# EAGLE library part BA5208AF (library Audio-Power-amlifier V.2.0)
3V-400mW BTL Power Audio Amplifier
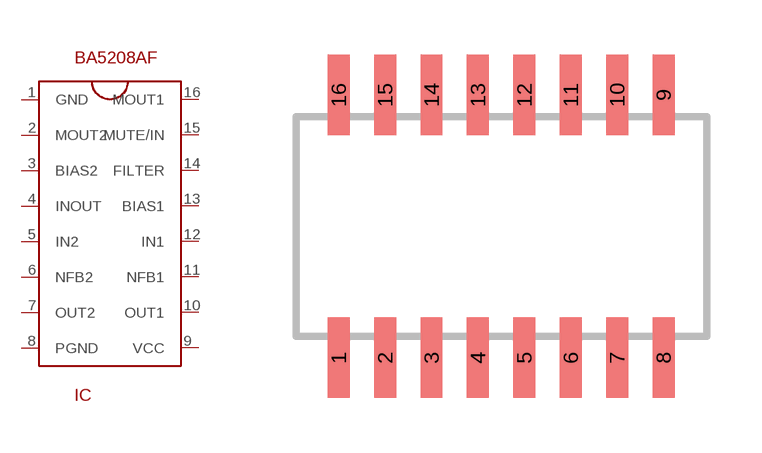
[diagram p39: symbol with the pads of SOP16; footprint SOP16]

Designator prefix IC

## BA5208AF  [SOP16]
1  GND  pwr
2  MOUT2  out
3  BIAS2
4  INOUT  out
5  IN2  in
6  NFB2
7  OUT2  out
8  PGND  pwr
9  VCC  pwr
10  OUT1  out
11  NFB1
12  IN1  in
13  BIAS1
14  FILTER
15  MUTE/IN  in
16  MOUT1  out

## Footprint SOP16 (pad centres in mm)
smd 0.6 x 2.2: 1 -4.445,-3.6; 2 -3.175,-3.6; 3 -1.905,-3.6; 4 -0.635,-3.6; 5 0.635,-3.6; 6 1.905,-3.6; 7 3.175,-3.6; 8 4.445,-3.6; 9 4.445,3.6; 10 3.175,3.6; 11 1.905,3.6; 12 0.635,3.6; 13 -0.635,3.6; 14 -1.905,3.6; 15 -3.175,3.6; 16 -4.445,3.6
